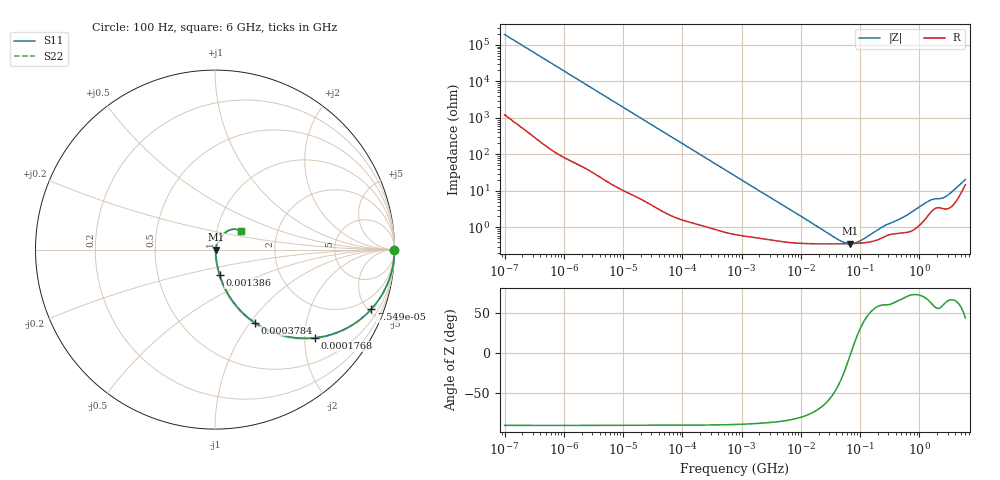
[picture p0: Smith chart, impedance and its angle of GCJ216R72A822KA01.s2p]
!Murata Part Number: GCJ216R72A822KA01
!These Parameters are Measured in Series Mode Connection
!Data Generated on Mar 13, 2026
!  o--ll--o
!Port1  Port2
!  o------o
!Operation Temp=25[degC], DC Bias Voltage=0[V]
!Freq. Start=100[Hz] Stop=6[GHz] 401[Steps]
# Hz S RI R 50
!Freq.(Hz) S11(Real) S11(Imag) S21(Real) S21(Imag) S12(Real) S12(Imag) S22(Real) S22(Imag)
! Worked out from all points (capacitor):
!   401 points, 100 Hz to 6 GHz, reference 50 ohm
!   read as one part in series: C = 8.2 nF near 109 Hz
!   lowest |Z| = 361 mohm at 68.17 MHz (marker M1)
!   series resonance near 69.97 MHz, so ESL is about 630 pH
!   S11 on the Smith chart (normalised r, x): 100 Hz: open; 75.5 kHz: 1.04, -5.24; 176.8 kHz: 1.02, -2.24; 378.4 kHz: 1.02, -1.05; 1.386 MHz: 1.01, -0.29; 6 GHz: 1.30, +0.28
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100  1 -0.000516  3.5e-06 0.000516  3.5e-06 0.000516  1 -0.000516
2008  0.9998 -0.0103  0.000155 0.0103  0.000155 0.0103  0.9998 -0.0103
12592  0.9956 -0.0638  0.00444 0.0638  0.00444 0.0638  0.9956 -0.0638
40335  0.9587 -0.1957  0.0413 0.1957  0.0413 0.1957  0.9587 -0.1957
75495  0.8709 -0.3317  0.1291 0.3317  0.1291 0.3317  0.8709 -0.3317
112960  0.7524 -0.4274  0.2476 0.4274  0.2476 0.4274  0.7524 -0.4274
176758  0.5565 -0.4914  0.4435 0.4914  0.4435 0.4914  0.5565 -0.4914
252896  0.3831 -0.4796  0.6169 0.4796  0.6169 0.4796  0.3831 -0.4796
378399  0.2206 -0.4066  0.7794 0.4066  0.7794 0.4066  0.2206 -0.4066
774597  0.0677 -0.2391  0.9323 0.2391  0.9323 0.2391  0.0677 -0.2391
1386327  0.0257 -0.1403  0.9743 0.1403  0.9743 0.1403  0.0257 -0.1403
3712478  0.00726 -0.054  0.9927 0.054  0.9927 0.054  0.00726 -0.054
1.555665e7  0.00373 -0.0125  0.9963 0.0125  0.9963 0.0125  0.00373 -0.0125
4.35672e7  0.00355 -0.00287  0.9964 0.00287  0.9964 0.00287  0.00355 -0.00287
6.817316e7  0.00359 -0.000151  0.9964 0.000151  0.9964 0.000151  0.00359 -0.000151
1.020051e8  0.00372 0.00227  0.9963 -0.00227  0.9963 -0.00227  0.00372 0.00227
3.124326e8  0.00643 0.011  0.9936 -0.011  0.9936 -0.011  0.00643 0.011
5.847788e8  0.00756 0.0191  0.9924 -0.0191  0.9924 -0.0191  0.00756 0.0191
1.431855e9  0.0236 0.0459  0.9764 -0.0459  0.9764 -0.0459  0.0236 0.0459
2.679998e9  0.0344 0.0557  0.9656 -0.0557  0.9656 -0.0557  0.0344 0.0557
4.009986e9  0.0542 0.0925  0.9458 -0.0925  0.9458 -0.0925  0.0542 0.0925
6e9  0.1424 0.1056  0.8576 -0.1056  0.8576 -0.1056  0.1424 0.1056
